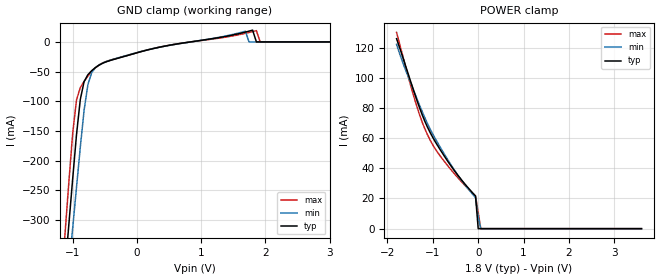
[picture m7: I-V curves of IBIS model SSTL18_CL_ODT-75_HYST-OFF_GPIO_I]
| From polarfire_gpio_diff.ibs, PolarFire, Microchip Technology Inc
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|   Model SSTL18_CL_ODT-75_HYST-OFF_GPIO_I
[Model]   SSTL18_CL_ODT-75_HYST-OFF_GPIO_I
Model_type   Input
Vinl =   0.775
Vinh =   1.025
|   typ   min   max
C_comp_pullup   2.605e-12   2.605e-12   2.76e-12
C_comp_pulldown  2.605e-12   2.605e-12   2.76e-12
[Temperature Range]  25C   100C   -40C
[Voltage Range]  1.8   1.71   1.89
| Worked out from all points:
|   POWER clamp passes 1 mA (typ) near -0.00 V on its own axis
[GND Clamp]
| Voltage   I(typ)   I(min)   I(max)
-1.8V     -1.26A     -1.229A    -1.314A
-1.122V   -382.2mA   -448.7mA   -320.1mA
-1.063V   -305.9mA   -380.7mA   -234.6mA
-1.004V   -229.8mA   -312.8mA   -153.2mA
-885.9mV  -96.92mA   -177.3mA   -77.03mA
-767.8mV  -55.27mA   -72.09mA   -57.55mA
-590.6mV  -38.92mA   -38.58mA   -38.65mA
1.688V    16.54mA    18.07mA    14.49mA
1.8V      19.81mA    0A         17.35mA
1.859V    0A         0A         18.96mA
1.918V    0A         0A         0A
3.6V      0A         0A         0A
[POWER Clamp]
| Voltage   I(typ)   I(min)   I(max)
-1.8V     125.9mA    122.1mA    130mA
-1.654V   112.8mA    109.3mA    113.4mA
-1.417V   90.97mA    91.23mA    87.4mA
-1.299V   80.67mA    82.28mA    76.05mA
-1.181V   71.48mA    73.82mA    66.51mA
-1.004V   60.6mA     62.79mA    55.6mA
-826.9mV  51.79mA    53.42mA    47.7mA
-472.5mV  36.3mA     36.45mA    34.56mA
-59.06mV  21.65mA    20.66mA    21.57mA
0V        0A         7.931mA    10.82mA
56.25mV   0A         0A         0A
3.6V      0A         0A         0A
